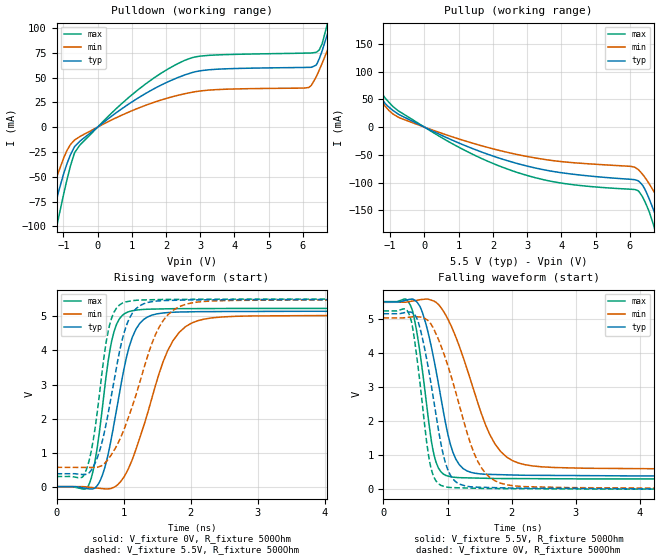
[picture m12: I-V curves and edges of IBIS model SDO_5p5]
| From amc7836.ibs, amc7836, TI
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|   Model
[Model]   SDO_5p5
Model_type   Output
Polarity   Non-Inverting
Vmeas = 2.75
Vref = 0
Cref = 1pF
Rref = 100000
|   typ   min   max
C_comp   2.780pF   2.357pF   3.166pF
[Voltage Range]   5.5   5.49   5.51
[Temperature Range]   27   125   -40
[Pullup Reference]   5.5   5.49   5.51
[Pulldown Reference]   0   0   0
[Power Clamp Reference]   5.5   5.49   5.51
[GND Clamp Reference]   0   0   0
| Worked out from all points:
|   slope of the pulldown table from 0 to 0.825 V, typ, clamps not added: 38.8 ohm
|   slope of the pullup table from 0 to 0.825 V, typ, clamps not added: 34.7 ohm
|   falling waveform, V_fixture 5.5V, R_fixture 500Ohm: 20-80 % time 320ps typ, 552ps min, 221ps max; typ from 5.5 V to 0.378 V
|   rising waveform, V_fixture 0V, R_fixture 500Ohm: 20-80 % time 308ps typ, 498ps min, 214ps max; typ from 0 V to 5.16 V
|   rising waveform, V_fixture 5.5V, R_fixture 500Ohm: 20-80 % time 310ps typ, 506ps min, 216ps max; typ from 0.378 V to 5.5 V
|   falling waveform, V_fixture 0V, R_fixture 500Ohm: 20-80 % time 288ps typ, 492ps min, 200ps max; typ from 5.16 V to 0 V
[Pulldown]
|   Voltage   I(typ)   I(min)   I(max)
-5.5V     -888.8mA   -641.4mA   -1.134A
-2.535V   -315.1mA   -218.8mA   -413.3mA
-1.375V   -101.7mA   -69.84mA   -135.7mA
-1.226V   -77.61mA   -53.82mA   -105.8mA
-797.5mV  -28.13mA   -17.73mA   -39.54mA
-517mV    -14.13mA   -9.502mA   -18.02mA
2.552V    52.69mA    33.72mA    67.43mA
6.165V    60.23mA    39.92mA    74.67mA
6.479V    69.03mA    57.65mA    77.95mA
6.71V     93.12mA    76.91mA    103.4mA
7.056V    133.5mA    107.7mA    154.4mA
11V       366.1mA    293.7mA    432mA
[Pullup]
|   Voltage   I(typ)   I(min)   I(max)
-5.5V     297.6mA    253.2mA    343.1mA
-3.586V   224.4mA    190.5mA    260.5mA
-2.794V   186mA      157.1mA    216.5mA
-2.167V   141.1mA    119.3mA    165.6mA
-1.375V   62.1mA     56.22mA    71.11mA
-764.5mV  23.41mA    17.92mA    29.35mA
2.717V    -65.64mA   -49.42mA   -81.75mA
6.231V    -96.32mA   -75.68mA   -114.2mA
6.726V    -154.4mA   -118.4mA   -183.6mA
6.891V    -182.4mA   -136.5mA   -220.9mA
8.079V    -403.7mA   -288.3mA   -507.7mA
11V       -973.3mA   -711.1mA   -1.222A
[Ramp]
R_load = 500
|   typ   min   max
dV/dt_r   3.09283/3.0821e-10   3.02018/4.97905e-10   3.14221/2.14447e-10
dV/dt_f   3.07308/3.20053e-10   2.95354/5.52349e-10   3.12777/2.21425e-10
[Falling Waveform]
V_fixture = 5.5V
V_fixture_min = 5.49V
V_fixture_max = 5.51V
R_fixture = 500Ohm
C_fixture = 0F
|   Time   V(typ)   V(min)   V(max)
0s        5.5V       5.49V      5.51V
386.6ps   5.569V     5.506V     5.516V
468.9ps   5.575V     5.533V     5.13V
586.5ps   5.3V       5.572V     3.789V
794ps     3.748V     5.521V     967.2mV
1.066ns   1.188V     4.758V     358.6mV
1.301ns   538.1mV    3.551V     332.8mV
1.736ns   430.2mV    1.339V     313.5mV
2.327ns   407.2mV    682.1mV    308.5mV
20ns      378.2mV    567.4mV    297.1mV
[Rising Waveform]
V_fixture = 0V
V_fixture_min = 0V
V_fixture_max = 0V
R_fixture = 500Ohm
C_fixture = 0F
|   Time   V(typ)   V(min)   V(max)
0s        1.063uV    -17.68uV   403.6nV
468.9ps   -59.67mV   -14.27mV   7.453mV
557.6ps   -52.86mV   -32.67mV   579.5mV
654.3ps   191.4mV    -52.72mV   1.84V
857.6ps   1.849V     -16.01mV   4.559V
1.041ns   3.784V     409.5mV    5.109V
1.186ns   4.631V     1.107V     5.186V
1.736ns   5.122V     4.285V     5.227V
2.327ns   5.142V     4.959V     5.232V
20ns      5.155V     5.034V     5.237V
[Rising Waveform]
V_fixture = 5.5V
V_fixture_min = 5.49V
V_fixture_max = 5.51V
R_fixture = 500Ohm
C_fixture = 0F
|   Time   V(typ)   V(min)   V(max)
0s        378.2mV    567.4mV    297.1mV
386.6ps   355.1mV    563.6mV    281.5mV
482.7ps   401mV      562.6mV    739.9mV
567.2ps   659mV      561.8mV    1.618V
794ps     2.41V      869.5mV    4.769V
965.3ps   4.204V     1.483V     5.371V
1.12ns    5.061V     2.303V     5.461V
1.59ns    5.466V     4.877V     5.499V
2.208ns   5.487V     5.441V     5.504V
20ns      5.5V       5.49V      5.51V
[Falling Waveform]
|Gnd
V_fixture = 0V
V_fixture_min = 0V
V_fixture_max = 0V
R_fixture = 500Ohm
C_fixture = 0F
|   Time   V(typ)   V(min)   V(max)
0s        5.155V     5.034V     5.237V
371.1ps   5.202V     5.046V     5.246V
437.8ps   5.197V     5.06V      4.918V
532ps     4.972V     5.064V     3.721V
747.5ps   3.039V     4.833V     579.1mV
977ps     717.6mV    3.79V      64.71mV
1.129ns   213.9mV    2.84V      42.66mV
1.474ns   57.62mV    806.2mV    25.09mV
2.016ns   32.31mV    102.1mV    14.88mV
20ns      -50.64uV   135.5uV    414.4nV
